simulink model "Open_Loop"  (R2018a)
settings: Solver=VariableStepAuto  StartTime=0.0  StopTime=50  FixedStep=Ts  MaxStep=0.05  RelTol=1e-3  EnableMultiTasking=on
InitFcn:
  | init
undefined symbols (not defined in the file or in its folder): Aa, Av, Ba, Bv, Ca, Cv, Da, Dv, Kmix, Kq

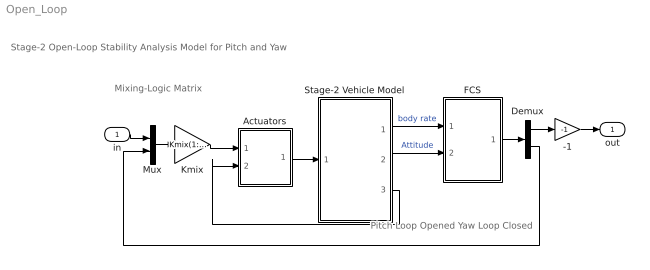
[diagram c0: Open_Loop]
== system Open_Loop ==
  note: Pitch Loop Opened Yaw Loop Closed
  note: Stage-2 Open-Loop Stability Analysis Model for Pitch and Yaw
  note: Mixing-Logic Matrix
  in : Inport
  -1 : Gain  Gain=-1
  Actuators : Subsystem
  Demux : Demux  Outputs=2
  FCS : Subsystem
  Kmix : Gain  Gain=Kmix(1:2,2:3)  Multiplication=Matrix(K*u)
  Mux : Mux  Inputs=2
  Stage-2 Vehicle Model : Subsystem
  out : Outport
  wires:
  Stage-2 Vehicle Model/1(Wb) -> FCS/1(rate)  "body rate"
  Stage-2 Vehicle Model/2(atti) -> FCS/2(atter)  "Attitude"
  FCS/1(DQ,DR) -> Demux/1
  Actuators/1(del) -> Stage-2 Vehicle Model/1(dy,dz)
  Kmix/1 -> Actuators/1(dc)
  Stage-2 Vehicle Model/3(TL) -> Actuators/2(TL)
  Mux/1 -> Kmix/1
  -1/1 -> out/1
  in/1 -> Mux/1
  Demux/1 -> -1/1
  Demux/2 -> Mux/2

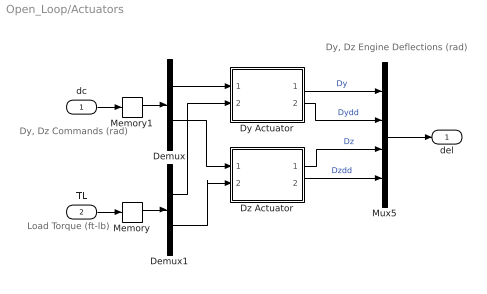
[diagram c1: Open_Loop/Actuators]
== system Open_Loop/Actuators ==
  note: Dy, Dz Engine Deflections (rad)
  note: Load Torque (ft-lb)
  note: Dy, Dz Commands (rad)
  dc : Inport
  TL : Inport  Port=2
  Demux : Demux  Outputs=2
  Demux1 : Demux  Outputs=2
  Dy Actuator : Subsystem
  Dz Actuator : Subsystem
  Memory : Memory
  Memory1 : Memory
  Mux5 : Mux
  del : Outport
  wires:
  Demux1/1 -> Dy Actuator/2(TL)
  Mux5/1 -> del/1
  Demux1/2 -> Dz Actuator/2(TL)
  Demux/2 -> Dz Actuator/1(dc)
  Dy Actuator/1(del) -> Mux5/1  "Dy"
  Dy Actuator/2(ddd) -> Mux5/2  "Dydd"
  Demux/1 -> Dy Actuator/1(dc)
  Dz Actuator/1(del) -> Mux5/3  "Dz"
  Dz Actuator/2(ddd) -> Mux5/4  "Dzdd"
  dc/1 -> Memory1/1
  TL/1 -> Memory/1
  Memory/1 -> Demux1/1
  Memory1/1 -> Demux/1

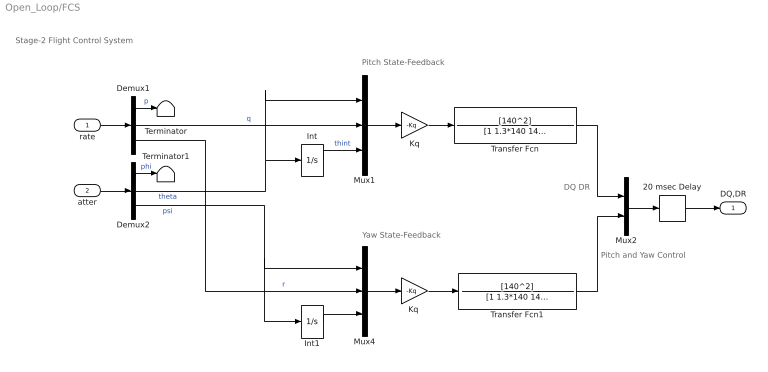
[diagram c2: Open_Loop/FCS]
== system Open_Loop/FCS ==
  note: DQ DR
  note: Pitch State-Feedback
  note: Yaw State-Feedback
  note: Pitch and Yaw Control
  note: Stage-2 Flight Control System
  rate : Inport
  atter : Inport  Port=2
  20 msec Delay : TransportDelay  DelayTime="[1  1]*0.020"  InitialOutput=[0 0]  PadeOrder=2
  Demux1 : Demux  Outputs=3
  Demux2 : Demux  Outputs=3
  Int : Integrator
  Int1 : Integrator
  Kq : Gain  Gain=-Kq  Multiplication=Matrix(K*u)
  "Kq " : Gain  Gain=-Kq  Multiplication=Matrix(K*u)
  Mux1 : Mux  Inputs=3
  Mux2 : Mux  Inputs=2
  Mux4 : Mux  Inputs=3
  Terminator : Terminator
  Terminator1 : Terminator
  Transfer Fcn : TransferFcn  Numerator=[140^2]  Denominator=[1 1.3*140 140^2]
  Transfer Fcn1 : TransferFcn  Numerator=[140^2]  Denominator=[1 1.3*140 140^2]
  DQ,DR : Outport
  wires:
  Mux2/1 -> 20 msec Delay/1
  rate/1 -> Demux1/1
  Kq/1 -> Transfer Fcn/1
  Demux2/2 -> Mux1/1, Int/1  "theta"
  Demux1/2 -> Mux1/2  "q"
  Int/1 -> Mux1/3  "thint"
  Int1/1 -> Mux4/3
  Demux1/3 -> Mux4/2  "r"
  Demux2/3 -> Int1/1, Mux4/1  "psi"
  atter/1 -> Demux2/1
  Mux1/1 -> Kq/1
  Transfer Fcn/1 -> Mux2/1
  Transfer Fcn1/1 -> Mux2/2
  Mux4/1 -> "Kq "/1
  "Kq "/1 -> Transfer Fcn1/1
  Demux1/1 -> Terminator/1  "p"
  Demux2/1 -> Terminator1/1  "phi"
  20 msec Delay/1 -> DQ,DR/1

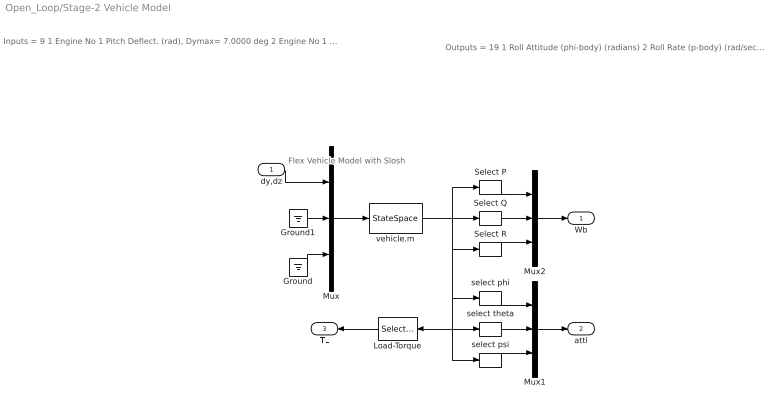
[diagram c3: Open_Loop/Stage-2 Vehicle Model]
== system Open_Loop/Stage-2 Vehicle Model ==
  note: Inputs = 9 1 Engine No 1 Pitch Deflect. (rad), Dymax= 7.0000 deg 2 Engine No 1 Pitch Acceleration (rad/sec^2) 3 Engine No 1 Yaw Deflect. (rad), Dzmax= 7.0000 deg 4 Engine No 1 Yaw Acceleration (rad/sec^2) 5 Throttle Input dTh/Th for Engine No 2 (-) 6 Throttle Input dTh/Th for Engine No 3 (-) 7 Throttle Input dTh/Th for Engine No 4 (-) 8 Throttle Input dTh/Th for Engine No 5 (-) 9 Wind Gust Azim, Elev Angles=( 45.0 90.0) (deg)
  note: Outputs = 19 1 Roll Attitude (phi-body) (radians) 2 Roll Rate (p-body) (rad/sec) 3 Pitch Attitude (thet-bdy) (radians) 4 Pitch Rate (q-body) (rad/sec) 5 Yaw Attitude (psi-body) (radians) 6 Yaw Rate (r-body) (rad/sec) 7 Angle of attack, alfa, (radians) 8 Angle of sideslip, beta, (radian) 9 Change in Altitude, delta-h, (feet) 10 Forward Acceleration (V-dot) (ft/sec) 11 Cross Range Velocity (Vcr) (ft/sec) 12 Rate-Gyro # 1, Roll Rate (Body) (rad/sec) 13 Rate-Gyro # 2, Pitch Rate (Body) (rad/sec) 14 Rate-Gyro # 3, Yaw Rate (Body) (rad/sec) 15 CG Acceleration along X axis, (ft/sec^2) 16 CG Acceleration along Y axis, (ft/sec^2) 17 CG Acceleration along Z axis, (ft/sec^2) 18 Ptch Load-Torque Tly for Engine: 1,(ft-lb) 19 Yaw Load-Torque Tlz for Engine: 1,(ft-lb)
  note: Flex Vehicle Model with Slosh
  dy,dz : Inport
  Ground : Ground
  Ground1 : Ground
  Load-Torque : Selector  InputPortWidth=19  IndexOptions=Index vector (dialog)  Indices=[18, 19]  OutputSizes=1
  Mux : Mux  Inputs=[4,4,1]
  Mux1 : Mux  Inputs=3
  Mux2 : Mux  Inputs=3
  Select P : Selector  InputPortWidth=19  IndexOptions=Index vector (dialog)  Indices=[12]  OutputSizes=1
  Select Q : Selector  InputPortWidth=19  IndexOptions=Index vector (dialog)  Indices=[13]  OutputSizes=1
  Select R : Selector  InputPortWidth=19  IndexOptions=Index vector (dialog)  Indices=[14]  OutputSizes=1
  select phi : Selector  InputPortWidth=19  IndexOptions=Index vector (dialog)  Indices=[1]  OutputSizes=1
  select psi : Selector  InputPortWidth=19  IndexOptions=Index vector (dialog)  Indices=[5]  OutputSizes=1
  select theta : Selector  InputPortWidth=19  IndexOptions=Index vector (dialog)  Indices=[3]  OutputSizes=1
  vehicle.m : StateSpace  A=Av  B=Bv  C=Cv  D=Dv  InitialCondition=0
  Wb : Outport
  atti : Outport  Port=2
  TL : Outport  Port=3
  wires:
  Load-Torque/1 -> TL/1
  Ground/1 -> Mux/3
  dy,dz/1 -> Mux/1
  Select P/1 -> Mux2/1
  Mux/1 -> vehicle.m/1
  Select R/1 -> Mux2/3
  Mux1/1 -> atti/1
  select theta/1 -> Mux1/2
  Select Q/1 -> Mux2/2
  vehicle.m/1 -> Select Q/1, Select P/1, Select R/1, select phi/1, select psi/1, Load-Torque/1, select theta/1
  select phi/1 -> Mux1/1
  select psi/1 -> Mux1/3
  Mux2/1 -> Wb/1
  Ground1/1 -> Mux/2

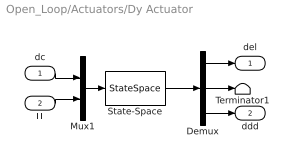
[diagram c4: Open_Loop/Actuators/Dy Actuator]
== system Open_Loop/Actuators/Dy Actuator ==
  dc : Inport
  TL : Inport  Port=2
  Demux : Demux  Outputs=3
  Mux1 : Mux  Inputs=2
  State-Space : StateSpace  A=Aa  B=Ba  C=Ca  D=Da  InitialCondition=0
  Terminator1 : Terminator
  del : Outport
  ddd : Outport  Port=2
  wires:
  Demux/1 -> del/1
  Demux/2 -> Terminator1/1
  Demux/3 -> ddd/1
  Mux1/1 -> State-Space/1
  State-Space/1 -> Demux/1
  dc/1 -> Mux1/1
  TL/1 -> Mux1/2

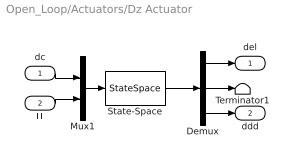
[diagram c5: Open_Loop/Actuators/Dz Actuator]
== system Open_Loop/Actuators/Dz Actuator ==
  dc : Inport
  TL : Inport  Port=2
  Demux : Demux  Outputs=3
  Mux1 : Mux  Inputs=2
  State-Space : StateSpace  A=Aa  B=Ba  C=Ca  D=Da  InitialCondition=0
  Terminator1 : Terminator
  del : Outport
  ddd : Outport  Port=2
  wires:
  Demux/1 -> del/1
  Demux/2 -> Terminator1/1
  Demux/3 -> ddd/1
  Mux1/1 -> State-Space/1
  State-Space/1 -> Demux/1
  dc/1 -> Mux1/1
  TL/1 -> Mux1/2
